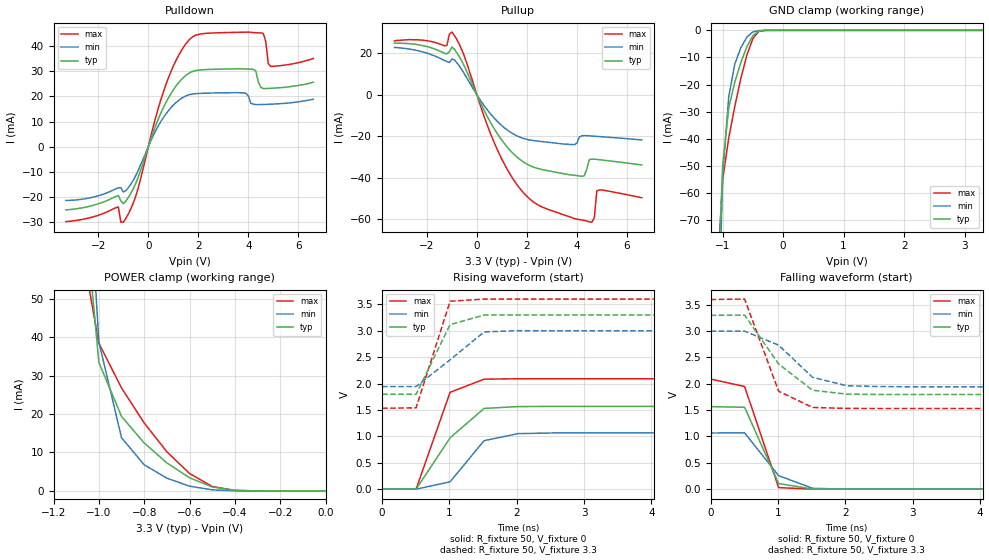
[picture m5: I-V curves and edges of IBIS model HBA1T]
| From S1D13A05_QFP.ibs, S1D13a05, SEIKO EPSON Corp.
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[Model]   HBA1T
Model_type I/O
Enable Active-Low
Polarity Non-Inverting
Vinh=2.0
Vinl=0.8
Vref=0
Vmeas=1.65
Rref=500
Cref=100pf
C_comp   5p   4p   6p
[Temperature Range] 25   85   -40
[Voltage Range]   3.3   3.0   3.6
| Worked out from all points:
|   slope of the pulldown table from 0 to 0.495 V, typ, clamps not added: 37.3 ohm
|   slope of the pullup table from 0 to 0.495 V, typ, clamps not added: 40.4 ohm
|   GND clamp passes 1 mA (typ) near -0.44 V on its own axis
|   POWER clamp passes 1 mA (typ) near -0.50 V on its own axis
|   falling waveform, R_fixture 50, V_fixture 0: 20-80 % time 328ps typ, 462ps min, 330ps max; typ from 1.57 V to 0 V
|   falling waveform, R_fixture 50, V_fixture 3.3: 20-80 % time 622ps typ, 584ps min, 358ps max; typ from 3.3 V to 1.8 V
|   rising waveform, R_fixture 50, V_fixture 0: 20-80 % time 598ps typ, 414ps min, 345ps max; typ from 0 V to 1.57 V
|   rising waveform, R_fixture 50, V_fixture 3.3: 20-80 % time 345ps typ, 619ps min, 311ps max; typ from 1.8 V to 3.3 V
[Pullup]
-3.3V     24.95mA    22.87mA    26.05mA
-1.3V     20.04mA    16.56mA    23.66mA
-1V       23.11mA    17.29mA    30.31mA
-500mV    13.79mA    10.13mA    18.59mA
1V        -21.95mA   -14.91mA   -31.14mA
2.4V      -35.47mA   -22.32mA   -52.86mA
3.9V      -38.89mA   -24.04mA   -59.76mA
4.2V      -39.37mA   -19.82mA   -60.46mA
4.6V      -31.08mA   -19.92mA   -61.56mA
4.7V      -31.1mA    -20mA      -59.45mA
4.8V      -31.23mA   -20.09mA   -46.41mA
6.6V      -33.9mA    -21.81mA   -49.75mA
[Pulldown]
-3.3V     -25.21mA   -21.41mA   -29.88mA
-1.2V     -19.46mA   -16.43mA   -24.03mA
-1V       -22.72mA   -18.08mA   -30.1mA
-500mV    -14.53mA   -11.43mA   -19.62mA
800mV     19.37mA    14.28mA    27.3mA
1.8V      30.07mA    21mA       43.92mA
3.8V      30.97mA    21.44mA    45.6mA
4.2V      30.79mA    16.97mA    45.46mA
4.5V      23.66mA    16.78mA    45.32mA
4.7V      23.16mA    16.84mA    41.88mA
4.9V      23.24mA    16.91mA    31.95mA
6.6V      25.67mA    18.9mA     35.13mA
[GND Clamp]
-3.3V     -4.101A    -3.648A    -4.786A
-1.1V     -105.4mA   -133.5mA   -94.8mA
-1V       -49.55mA   -53.37mA   -54.84mA
-900mV    -28.46mA   -24.39mA   -39.63mA
-800mV    -19.05mA   -12.36mA   -27.97mA
-700mV    -11.87mA   -6.396mA   -17.69mA
-600mV    -6.023mA   -2.492mA   -9.098mA
-500mV    -1.964mA   -559.2uA   -2.968mA
-400mV    -291.4uA   -72.87uA   -373.1uA
-300mV    -21.59uA   -6.634uA   -18.01uA
3.3V      1.197nA    2.93uA     77.17pA
[POWER Clamp]
-3.3V     4.135A     3.69A      4.781A
-1.1V     97.06mA    138.5mA    71.54mA
-1V       33.42mA    38.72mA    38.38mA
-900mV    19.35mA    13.82mA    26.76mA
-800mV    12.46mA    6.789mA    17.66mA
-700mV    7.279mA    3.31mA     10.17mA
-600mV    3.412mA    1.231mA    4.534mA
-500mV    1.036mA    277uA      1.153mA
-400mV    155.5uA    36.16uA    108uA
0V        1.197nA    2.433nA    175.4pA
[Falling Waveform]
R_fixture=50
V_fixture=0
V_fixture_min=0
V_fixture_max=0
0s        1.567V     1.066V     2.091V
505.1ps   1.554V     1.068V     1.949V
1.01ns    105.9mV    256.2mV    29.47mV
1.515ns   1.543mV    16.07mV    -343.1uV
2.02ns    153.9uV    -253.4uV   123.4uV
50ns      -3.352uV   -4.614uV   2.319uV
[Falling Waveform]
R_fixture=50
V_fixture=3.3
V_fixture_min=3.0
V_fixture_max=3.6
0s        3.3V       3V         3.6V
505.1ps   3.303V     3V         3.609V
1.01ns    2.375V     2.733V     1.859V
1.515ns   1.878V     2.122V     1.551V
2.02ns    1.804V     1.964V     1.533V
2.525ns   1.797V     1.947V     1.532V
3.03ns    1.797V     1.943V     1.532V
50ns      1.797V     1.943V     1.532V
[Rising Waveform]
R_fixture=50
V_fixture=0
V_fixture_min=0
V_fixture_max=0
0s        0V         0V         0V
505.1ps   -11.84uV   -7.236uV   1.074mV
1.01ns    971.8mV    139mV      1.835V
1.515ns   1.529V     918.9mV    2.083V
2.02ns    1.564V     1.052V     2.091V
3.03ns    1.567V     1.066V     2.091V
50ns      1.567V     1.066V     2.091V
[Rising Waveform]
R_fixture=50
V_fixture=3.3
V_fixture_min=3.0
V_fixture_max=3.6
0s        1.797V     1.943V     1.532V
505.1ps   1.797V     1.944V     1.54V
1.01ns    3.117V     2.451V     3.559V
1.515ns   3.297V     2.978V     3.6V
2.02ns    3.3V       3.002V     3.6V
50ns      3.3V       3V         3.6V
[Ramp]
R_load=50
dV/dt_r   9.403E-1/3.279E-10   6.398E-1/3.872E-10   1.254E+0/2.508E-10
dV/dt_f   9.017E-1/4.207E-10   6.340E-1/4.843E-10   1.241E+0/3.294E-10
